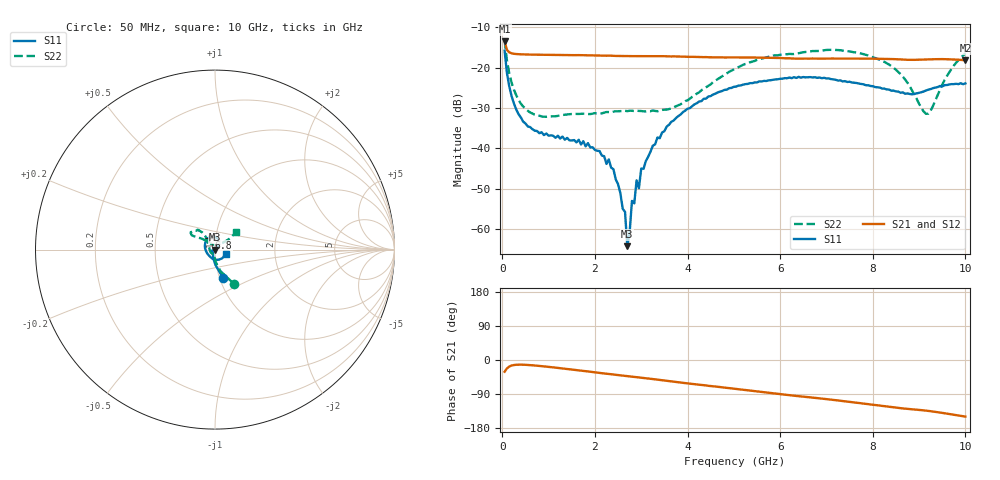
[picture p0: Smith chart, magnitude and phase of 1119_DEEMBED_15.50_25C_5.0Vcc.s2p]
!Hittite Microwave Corp.
!Digital Attenuator/PhaseShifter Rev 1.4.0
!Filename: C:\DATA\DATA\1119_DEEMBED_15.50_25C_5.0Vcc.s2p
!VNA ID: Agilent Technologies,N5224A,MY51441122,A.10.45.03
!Device type:
!2 Port Calibration.
!Temp(C): 25
!Lot Number:
!Serial Number:
!Operator:
!Misc:
!Attenuator:  15.500
# GHZ S DB R 50.0
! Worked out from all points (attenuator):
!   200 points, 50 MHz to 10 GHz, reference 50 ohm
!   highest |S21| = -13.47 dB at 50 MHz (marker M1); lowest = -18.2 dB at 10 GHz (marker M2)
!   lowest |S11| = -64.3 dB at 2.7 GHz (marker M3), VSWR 1.00, Z = 50 - j0.0397 ohm
!   |S11| at or under -10 dB: start of sweep to end of sweep
!   |S22| runs from -32.2 to -13.3 dB; largest |S21 - S12| = 0.00049
!   S11 on the Smith chart (normalised r, x): 50 MHz: 1.04, -0.33; 6.8 GHz: 0.93, +0.12; 10 GHz: 1.13, -0.05
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0.05  -15.80 -74.2  -13.47 -31.0  -13.47 -31.1  -13.26 -61.2
0.2  -27.05 -102.2  -16.44 -14.7  -16.44 -14.7  -23.70 -87.2
0.45  -33.39 -124.8  -16.72 -12.4  -16.73 -12.4  -29.63 -97.7
0.9  -36.74 -151.2  -16.82 -16.8  -16.82 -16.9  -32.19 -107.2
1.75  -38.26 -164.6  -16.92 -28.7  -16.92 -28.7  -31.44 -116.5
2.4  -45.23 178.0  -17.08 -38.5  -17.08 -38.5  -30.94 -133.6
2.65  -55.78 140.8  -17.15 -41.8  -17.15 -41.9  -30.72 -141.4
2.7  -64.31 -40.7  -17.14 -42.5  -17.15 -42.5  -30.81 -142.3
2.75  -60.90 65.5  -17.16 -43.1  -17.17 -43.2  -30.69 -144.5
2.8  -53.08 16.9  -17.15 -43.8  -17.16 -43.8  -30.71 -146.8
2.85  -53.68 27.3  -17.15 -44.6  -17.16 -44.6  -30.79 -148.8
2.9  -47.97 22.9  -17.17 -45.1  -17.18 -45.2  -30.68 -151.4
2.95  -49.94 21.3  -17.15 -45.8  -17.16 -45.8  -30.75 -153.7
3  -45.04 28.3  -17.15 -46.6  -17.16 -46.7  -30.77 -156.5
3.4  -37.53 43.8  -17.17 -52.5  -17.18 -52.5  -30.66 -176.7
4  -30.20 50.5  -17.33 -61.6  -17.34 -61.7  -28.12 149.4
5.05  -24.71 69.1  -17.47 -76.2  -17.49 -76.2  -20.13 125.5
6.7  -22.44 113.5  -17.75 -99.2  -17.77 -99.2  -15.89 139.8
6.8  -22.54 116.3  -17.77 -100.6  -17.79 -100.6  -15.89 141.1
8.35  -25.44 179.8  -17.86 -123.3  -17.86 -123.3  -19.23 143.0
9.2  -25.48 -101.4  -17.96 -134.3  -17.97 -134.4  -31.42 82.5
10  -23.91 -20.5  -18.17 -149.4  -18.18 -149.3  -16.46 39.7
